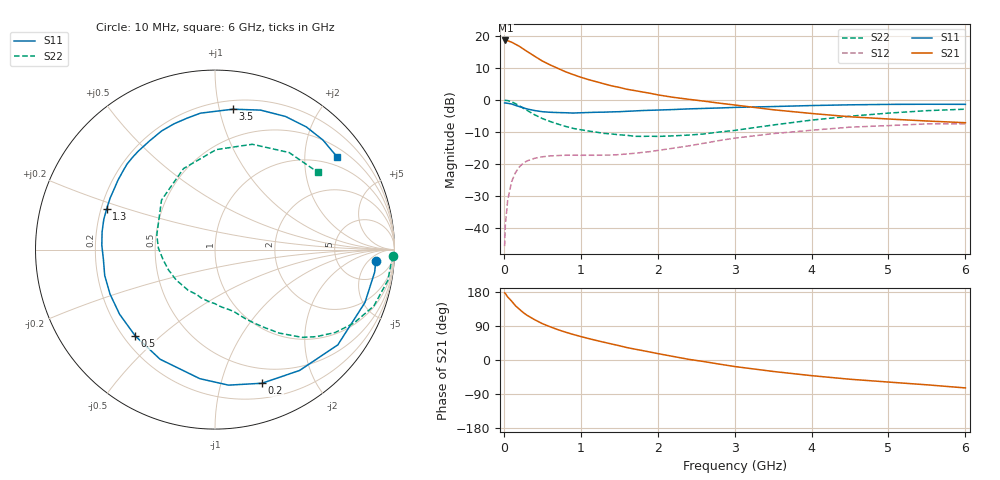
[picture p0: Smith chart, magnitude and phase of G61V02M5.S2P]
! SIEMENS Small Signal Semiconductors
! BFG193
! Si NPN RF Bipolar Junction Transistor in SOT223
! VCE = 1 V  IC = 2.5 mA
! Common Emitter S-Parameters:  August  1996
# GHz  S  MA  R  50
!  f  S11  S21  S12  S22
! GHz  MAG  ANG  MAG  ANG  MAG  ANG  MAG  ANG
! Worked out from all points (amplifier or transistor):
!   36 points, 10 MHz to 6 GHz, reference 50 ohm
!   highest |S21| = 18.6 dB at 20 MHz (marker M1)
!   |S21| within 3 dB of that: start of sweep to 274.9 MHz
!   unconditionally stable (mu >= 1): 1.289 GHz to 2.991 GHz
!   at 250 MHz: K = 0.22, MSG = 17.9 dB, |S12| = -19.8 dB
!   at 1.4 GHz: K = 1.07, MAG = 9.2 dB, |S12| = -17.2 dB
!   at 6 GHz: K = 1.00, MSG = 0.2 dB, |S12| = -7.5 dB
!   S11 on the Smith chart (normalised r, x): 10 MHz: 13, -8; 200 MHz: 0.34, -1.36; 500 MHz: 0.25, -0.42; 1.3 GHz: 0.22, +0.17; 3.5 GHz: 0.27, +1.10; 6 GHz: 0.73, +2.79
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0.01  0.898 -3.9  8.436 177.2  0.0052 91.2  0.9948 -2.1
0.02  0.8985 -8.0  8.497 175.6  0.0113 89.6  0.9853 -4.0
0.05  0.886 -19.4  8.399 166.3  0.0271 77.8  0.9781 -10.1
0.1  0.866 -37.8  8 155.7  0.0525 70.4  0.9394 -19.5
0.15  0.8219 -55.0  7.435 143.4  0.0729 60.1  0.8757 -27.9
0.2  0.7894 -70.6  6.901 134.4  0.0894 52.9  0.8134 -34.6
0.25  0.7589 -84.3  6.296 125.5  0.1023 46.2  0.745 -40.6
0.3  0.7241 -96.7  5.746 118.2  0.1114 41.2  0.6894 -45.2
0.4  0.6832 -116.6  4.82 106.4  0.1227 33.2  0.5871 -52.4
0.5  0.6548 -132.7  4.059 96.0  0.1294 27.1  0.5129 -57.7
0.6  0.6421 -145.9  3.536 87.8  0.1335 23.2  0.4618 -62.1
0.7  0.6353 -157.0  3.123 80.2  0.1353 20.5  0.4211 -66.2
0.9  0.6242 -175.0  2.493 67.5  0.1372 17.0  0.3598 -73.2
1.1  0.6369 171.0  2.079 56.7  0.1369 15.8  0.3272 -81.7
1.3  0.6449 159.3  1.789 46.9  0.1378 15.9  0.3008 -90.2
1.6  0.6647 144.4  1.468 32.8  0.1434 17.8  0.2803 -105.9
2.2  0.7075 120.8  1.1 9.4  0.1761 20.3  0.2748 -142.1
2.8  0.7491 101.8  0.892 -10.8  0.2322 15.8  0.3155 178.5
3.5  0.7886 82.7  0.703 -30.2  0.2981 1.8  0.4061 137.2
4.5  0.8394 62.1  0.546 -50.8  0.3757 -19.0  0.5572 89.3
5.5  0.8568 45.4  0.469 -65.5  0.4231 -44.1  0.6806 52.6
6  0.854 37.4  0.441 -73.7  0.4239 -58.0  0.7174 36.8
